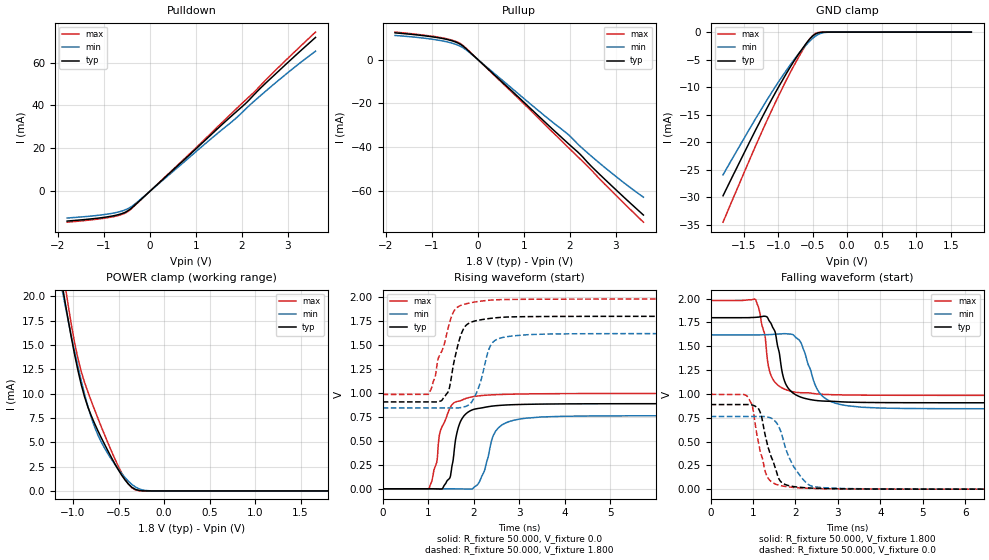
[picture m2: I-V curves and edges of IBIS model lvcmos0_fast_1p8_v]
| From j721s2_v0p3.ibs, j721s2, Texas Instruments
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|   fast_1p8_v
[Model]   lvcmos0_fast_1p8_v
Model_type I/O
Polarity   Non-Inverting
Enable   Active-High
Vinl = 0
Vinh = 0.8
Vmeas = 0.9
Vref = 1.8
Cref = 2pF
Rref = 100000
|   typ   min   max
C_comp   2.420pF   2.171pF   2.648pF
[Voltage Range]   1.8   1.62   1.98
[Temperature Range]   27   150   -40
[Pullup Reference]   1.8   1.62   1.98
[Pulldown Reference]   0   0   0
[Power Clamp Reference]   1.8   1.62   1.98
[GND Clamp Reference]   0   0   0
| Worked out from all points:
|   slope of the pulldown table from 0 to 0.27 V, typ, clamps not added: 50.8 ohm
|   slope of the pullup table from 0 to 0.27 V, typ, clamps not added: 51.4 ohm
|   GND clamp passes 1 mA (typ) near -0.52 V on its own axis
|   POWER clamp passes 1 mA (typ) near -0.42 V on its own axis
|   rising waveform, R_fixture 50.000, V_fixture 0.0: 20-80 % time 214ps typ, 296ps min, 308ps max; typ from 0 V to 0.888 V
|   rising waveform, R_fixture 50.000, V_fixture 1.800: 20-80 % time 251ps typ, 282ps min, 341ps max; typ from 0.906 V to 1.8 V
|   falling waveform, R_fixture 50.000, V_fixture 1.800: 20-80 % time 258ps typ, 400ps min, 247ps max; typ from 1.8 V to 0.906 V
|   falling waveform, R_fixture 50.000, V_fixture 0.0: 20-80 % time 332ps typ, 441ps min, 267ps max; typ from 0.888 V to 0 V
[Pulldown]
|Voltage   I(typ)   I(min)   I(max)
-1.8V     -13.91mA   -12.49mA   -14.44mA
-863mV    -11.73mA   -10.45mA   -12.14mA
-643mV    -10.64mA   -9.432mA   -11.05mA
-478mV    -9.09mA    -8.117mA   -9.44mA
-257mV    -5.071mA   -4.731mA   -5.198mA
1.286V    25.48mA    23.68mA    26.17mA
1.837V    36.29mA    33.41mA    37.59mA
2.057V    40.47mA    37.84mA    42.08mA
2.278V    45.32mA    42.22mA    46.45mA
2.718V    54.42mA    50.32mA    56.15mA
3.6V      71.7mA     65.29mA    74.2mA
[Pullup]
|Voltage   I(typ)   I(min)   I(max)
-1.8V     12.22mA    11.03mA    12.58mA
-1.249V   11.1mA     9.993mA    11.37mA
-808mV    9.795mA    8.672mA    10.06mA
-533mV    8.393mA    7.324mA    8.695mA
-367mV    6.813mA    5.929mA    7.149mA
-202mV    3.939mA    3.584mA    4.079mA
1.286V    -25.18mA   -22.83mA   -26.15mA
1.947V    -38.08mA   -33.96mA   -39.84mA
2.222V    -43.3mA    -39.66mA   -45.46mA
2.443V    -48.31mA   -43.75mA   -50.01mA
2.773V    -55.04mA   -49.61mA   -57.32mA
3.6V      -71.15mA   -62.97mA   -74.42mA
[GND_clamp]
|Voltage   I(typ)   I(min)   I(max)
-1.8V     -29.72mA   -25.92mA   -34.52mA
-1.318V   -17.54mA   -15.51mA   -20.38mA
-1.132V   -13.09mA   -11.7mA    -15.22mA
-984mV    -9.729mA   -8.822mA   -11.3mA
-798mV    -5.796mA   -5.487mA   -6.696mA
-612mV    -2.352mA   -2.574mA   -2.564mA
-538mV    -1.178mA   -1.582mA   -1.166mA
-464mV    -371.7uA   -771.3uA   -275.5uA
-353mV    -16.33uA   -129.3uA   -4.377uA
-241mV    -394.3nA   -10.85uA   -119.1nA
1.8V      0A         0A         0A
[POWER_clamp]
|Voltage   I(typ)   I(min)   I(max)
-1.8V     63.47mA    56.87mA    71.37mA
-1.132V   21.93mA    21.29mA    24mA
-1.095V   19.85mA    19.49mA    21.65mA
-1.058V   17.84mA    17.74mA    19.38mA
-984mV    14.08mA    14.39mA    15.3mA
-909mV    10.91mA    11.31mA    12.25mA
-761mV    6.887mA    6.531mA    8.298mA
-649mV    4.716mA    4.334mA    5.678mA
-464mV    1.599mA    1.771mA    1.827mA
-315mV    160.9uA    410.3uA    112.1uA
-130mV    304.4nA    7.74uA     148.3nA
1.8V      0A         0A         0A
[Ramp]
| variable   typ   min   max
dV/dt_r   0.533/0.214n   0.458/0.294n   0.597/0.308n
dV/dt_f   0.536/0.258n   0.466/0.398n   0.597/0.248n
R_load = 50.000
[Rising Waveform]
R_fixture= 50.000
V_fixture= 0.0
|time   V(typ)   V(min)   V(max)
0s        757nV      16.84uV    1.268uV
1.012ns   115.6uV    14.53uV    -447.6uV
1.309ns   453.1uV    19.11uV    653.2mV
1.485ns   127.5mV    -52.87uV   849.6mV
1.691ns   682.7mV    -1.271mV   916.9mV
1.956ns   821.4mV    -3.237mV   959mV
2.229ns   848.9mV    180.3mV    975.2mV
2.479ns   866.7mV    600.6mV    982mV
2.879ns   877.9mV    715.5mV    987.7mV
10ns      888.3mV    762.7mV    994.8mV
[Rising Waveform]
R_fixture= 50.000
V_fixture= 1.800
V_fixture_min= 1.620
V_fixture_max= 1.980
|time   V(typ)   V(min)   V(max)
0s        906.5mV    843.5mV    984.7mV
998ps     906.5mV    843.5mV    986mV
1.3ns     923.5mV    843.4mV    1.439V
1.456ns   1.035V     843.5mV    1.711V
1.571ns   1.336V     843.3mV    1.86V
1.746ns   1.64V      850.7mV    1.919V
1.911ns   1.732V     883.3mV    1.939V
2.367ns   1.778V     1.493V     1.969V
2.665ns   1.791V     1.582V     1.975V
10ns      1.8V       1.62V      1.98V
[Falling Waveform]
R_fixture= 50.000
V_fixture= 1.800
V_fixture_min= 1.620
V_fixture_max= 1.980
|time   V(typ)   V(min)   V(max)
0s        1.8V       1.62V      1.98V
1.06ns    1.804V     1.62V      1.99V
1.277ns   1.815V     1.621V     1.625V
1.335ns   1.806V     1.622V     1.374V
1.498ns   1.673V     1.626V     1.134V
1.727ns   1.156V     1.632V     1.053V
1.944ns   1.009V     1.621V     1.022V
2.554ns   928mV      1.019V     997.9mV
3.076ns   916.8mV    887.1mV    989.7mV
10ns      906.5mV    843.5mV    984.7mV
[Falling Waveform]
R_fixture= 50.000
V_fixture= 0.0
V_fixture_min= 0.0
V_fixture_max= 0.0
|time   V(typ)   V(min)   V(max)
0s        888.3mV    762.8mV    994.8mV
869ps     888.4mV    762.7mV    972.1mV
990ps     882.2mV    762.7mV    863.9mV
1.121ns   848.7mV    762.7mV    507.4mV
1.201ns   763.5mV    762.8mV    350.8mV
1.337ns   471.9mV    757.7mV    130mV
1.657ns   78.13mV    603.3mV    36.22mV
1.959ns   27.14mV    237.1mV    18.06mV
2.473ns   9.294mV    23.97mV    6.609mV
10ns      39.84uV    100uV      23.91uV
